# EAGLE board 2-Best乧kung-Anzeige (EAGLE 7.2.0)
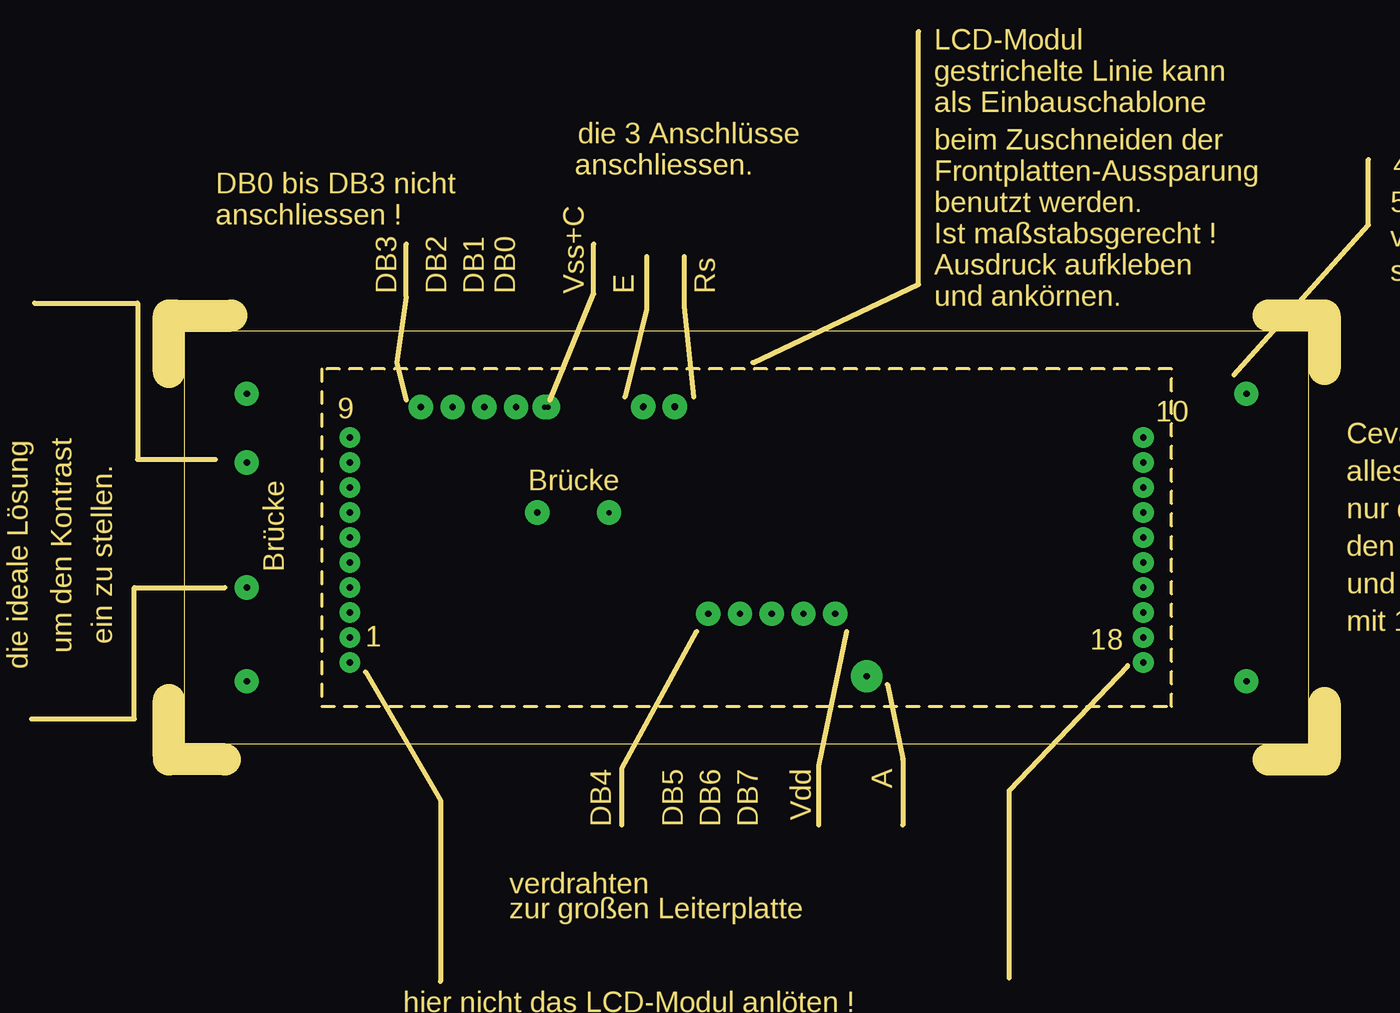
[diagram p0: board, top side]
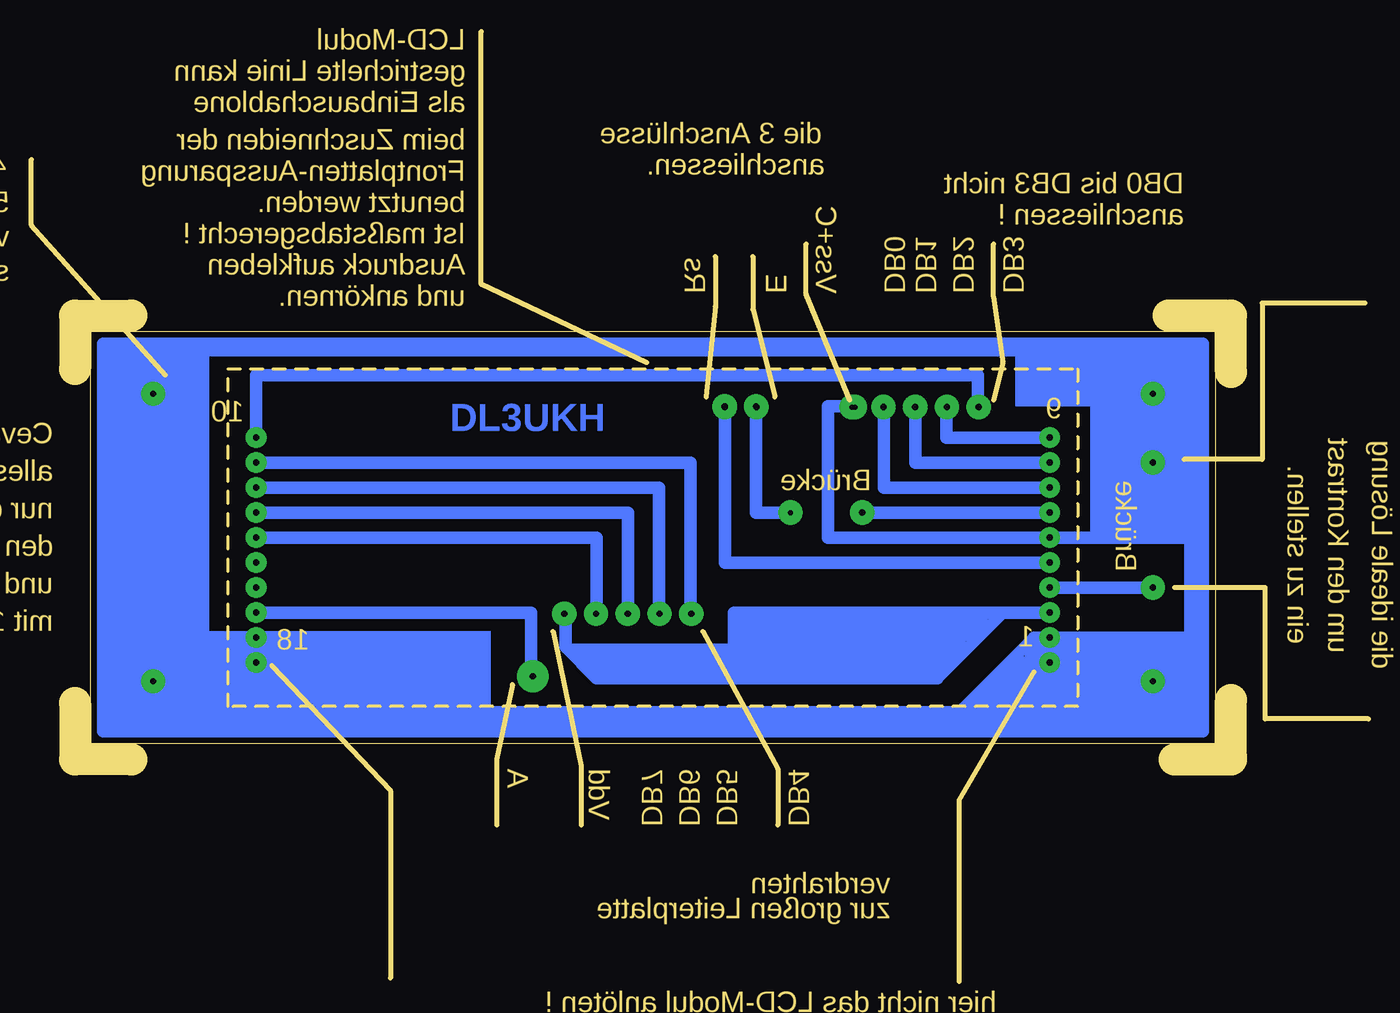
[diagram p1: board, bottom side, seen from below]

Size 107 x 76 mm. Coordinates in mm from the lower left corner, seen from the top.
Outline: 46 segments
Copper layers (1*16): Top 0.035mm / dielectric 1.5mm / Bottom 0.035mm
Design rules "default": minimum track width 10mil, minimum drill 24mil, track to track 8mil, track to pad 8mil, pad to pad 8mil, via to via 8mil, smd to smd 8mil, copper to edge 40mil, drill to drill 8mil, minimum pad ring 10mil, minimum via ring 8mil, stop-mask expansion 4mil, vias tented up to drill 0mil, thermal gap 10mil

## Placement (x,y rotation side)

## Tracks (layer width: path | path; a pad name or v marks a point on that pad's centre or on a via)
S$1  (via drill 0.4 pad 1.93)
  other vias: 17.25,24
S$2  (via drill 0.4 pad 1.68)
  Bottom 1.016: 31.75,21.5 27.75,25.5 v25.5,25.5 v25.5,27.5 26.75,27.5 33,21.25
S$3  (via drill 0.5 pad 1.68)
  Bottom 1.016: 31.75,21.5 27.75,25.5 v25.5,25.5 v25.5,27.5 26.75,27.5 33,21.25
S$4  (via drill 0.4 pad 1.93)
  other vias: 17.25,47
S$5  (via drill 0.4 pad 1.93)
  other vias: 97.25,24
S$6  (via drill 0.5 pad 1.68, 0.5 pad 1.93)
  Bottom 1.016: 54.25,29.5 54.25,41.5 v89,41.5
  other vias: 54.18,29.4
S$7  (via drill 0.5 pad 1.68)
  other vias: 25.5,31.5
S$8  (via drill 0.5 pad 1.93)
  other vias: 17.25,24
S$9  (via drill 0.4 pad 1.93)
  other vias: 97.25,47
S$10  (via drill 0.5 pad 1.93)
  other vias: 17.25,47
S$11  (via drill 0.5 pad 1.93)
  other vias: 97.25,24
S$12  (via drill 0.5 pad 1.93)
  other vias: 97.25,47
S$13
  Bottom 1.016: 93.25,20.25 93.25,51 98,51 | 21,51 21.25,51 | 21,51 98,51 | 98,51 101.25,51 101.25,20 13.25,20 13.25,51 21,51
S$14  (via drill 0.4 pad 1.68, 0.4 pad 1.93)
  Bottom 1.016: 17,31.5 v25.5,31.5 | 13.5,35.5 14.25,35.5 | 14.25,35.5 v25.5,35.5 43.25,35.5 43.25,46 41.25,46 | 31.75,21.5 27.75,25.5 v25.5,25.5 | 33,21.25 26.75,27.5 v25.5,27.5 | v25.5,25.5 20.5,25.5 | v25.5,27.5 v25.5,25.5 | 21.25,27.5 v25.5,27.5 | 21.25,27.5 14.25,27.5 | 14.25,27.5 13.75,27.5 | 21.25,20.25 21.25,27.5 | 14.25,35.5 14.25,27.5
  other vias: 41.34,45.94
S$15  (via drill 0.5 pad 1.68, 0.5 pad 1.93)
  Bottom 1.016: 56.75,29.5 56.75,39.5 v89,39.5
  other vias: 56.72,29.4
S$16  (via drill 0.4 pad 1.68)
  Bottom 1.016: v89,27.5 93.5,27.5
S$17  (via drill 0.4 pad 1.68)
  other vias: 89,31.5
S$18  (via drill 0.5 pad 1.68, 0.5 pad 1.93)
  Bottom 1.016: 59.25,29.5 59.25,37.5 v89,37.5
  other vias: 59.26,29.4
S$19  (via drill 0.5 pad 1.68, 0.5 pad 1.93)
  Bottom 1.016: 61.75,29.5 61.75,35.5 v89,35.5
  other vias: 61.8,29.4
S$20  (via drill 0.5 pad 1.68, 0.5 pad 1.93)
  Bottom 1.016: 31.25,45.75 31.25,48.5 35.75,48.5 | 35.75,48.5 36,48.5 | 35.75,48.5 89,48.5 v89,43.5
  other vias: 31.18,45.94
S$21  (via drill 0.5 pad 1.68)
  other vias: 25.5,31.5
S$22  (via drill 0.5 pad 1.93)
  other vias: 49,46 48.96,45.94
S$23  (via drill 0.4 pad 1.93)
  other vias: 17.25,24
S$24  (via drill 0.5 pad 1.68)
  other vias: 25.5,35.5
S$25  (via drill 0.4 pad 1.68)
  other vias: 89,33.5
S$26  (via drill 0.5 pad 1.93)
  other vias: 51.5,46 51.5,45.94
S$27  (via drill 0.5 pad 1.68, 0.5 pad 1.93)
  Bottom 1.016: v25.5,41.5 36.25,41.5 36.25,46
  other vias: 36.26,45.94
S$28  (via drill 0.5 pad 1.68)
  Bottom 1.016: v89,27.5 93.5,27.5
S$29  (via drill 0.5 pad 1.68)
  other vias: 89,31.5
S$30  (via drill 0.5 pad 1.68, 0.5 pad 1.93)
  Bottom 1.016: 38.75,46 38.75,39.5 v25.5,39.5
  other vias: 38.8,45.94
S$31  (via drill 0.5 pad 1.68)
  other vias: 89,33.5
S$32  (via drill 0.5 pad 1.68)
  other vias: 25.5,33.5
S$33  (via drill 0.5 pad 1.68, 0.5 pad 1.93)
  Bottom 1.016: 64.25,29.5 64.25,26.75 61.75,24.25 34.5,24.25 29.25,29.5 v25.5,29.5
  other vias: 64.34,29.4
S$34  (via drill 0.4 pad 1.93)
  other vias: 17.25,47
S$35  (via drill 0.5 pad 1.68, 0.5 pad 2.54)
  Bottom 1.016: 67,24.5 67,29.5 v89,29.5
  other vias: 66.86,24.4
S$36  (via drill 0.5 pad 1.68)
  other vias: 25.5,25.5
S$37  (via drill 0.5 pad 1.68)
  Bottom 1.016: v89,25.5 93.5,25.5
S$38  (via drill 0.5 pad 1.68, 0.5 pad 1.93)
  Bottom 1.016: v25.5,43.5 33.75,43.5 33.75,46
  other vias: 33.72,45.94
S$39  (via drill 0.5 pad 1.68, 0.5 pad 1.93)
  Bottom 1.016: v25.5,41.5 36.25,41.5 36.25,46
  other vias: 36.26,45.94
S$40  (via drill 0.5 pad 1.68, 0.5 pad 1.93)
  Bottom 1.016: 54.25,29.5 54.25,41.5 v89,41.5
  other vias: 54.18,29.4
S$41  (via drill 0.5 pad 1.68, 0.5 pad 1.93)
  Bottom 1.016: 56.75,29.5 56.75,39.5 v89,39.5
  other vias: 56.72,29.4
S$42  (via drill 0.5 pad 1.68, 0.5 pad 1.93)
  Bottom 1.016: 59.25,29.5 59.25,37.5 v89,37.5
  other vias: 59.26,29.4
S$43  (via drill 0.5 pad 1.68, 0.5 pad 1.93)
  Bottom 1.016: 61.75,29.5 61.75,35.5 v89,35.5
  other vias: 61.8,29.4
S$44  (via drill 0.5 pad 1.68, 0.5 pad 1.93)
  Bottom 1.016: 31.25,45.75 31.25,48.5 35.75,48.5 | 35.75,48.5 36,48.5 | 35.75,48.5 89,48.5 v89,43.5
  other vias: 31.18,45.94
S$45  (via drill 0.5 pad 1.68, 0.5 pad 1.93)
  Bottom 1.016: 38.75,46 38.75,39.5 v25.5,39.5
  other vias: 38.8,45.94
S$46  (via drill 0.5 pad 1.68, 0.5 pad 1.93)
  Bottom 1.016: 64.25,29.5 64.25,26.75 61.75,24.25 50.75,24.25 | 50.75,24.25 34.5,24.25 29.25,29.5 28.75,29.5 | 28.75,29.5 v25.5,29.5 | 28.75,29.5 50.75,29.5 50.75,24.25
  other vias: 64.34,29.4
S$47  (via drill 0.5 pad 1.68, 0.5 pad 2.54)
  Bottom 1.016: 67,24.5 67,29.5 v89,29.5
  other vias: 66.86,24.4
S$48  (via drill 0.5 pad 1.68)
  Bottom 1.016: v89,25.5 93.5,25.5
S$49  (via drill 0.5 pad 1.68, 0.5 pad 1.93)
  Bottom 1.016: v25.5,43.5 33.75,43.5 33.75,46
  other vias: 33.72,45.94
S$50  (via drill 0.5 pad 1.93)
  other vias: 49,46 48.96,45.94
S$51  (via drill 0.5 pad 1.93)
  Bottom 1.016: 51.5,34 v51.5,46
  other vias: 51.5,45.94
S$52  (via drill 0.4 pad 1.93)
  other vias: 97.25,24
S$53  (via drill 0.5 pad 1.68)
  other vias: 25.5,33.5 25.5,33.5
S$54  (via drill 0.5 pad 1.68)
  other vias: 25.5,37.5
S$55  (via drill 0.4 pad 1.93)
  other vias: 97.25,47
S$56
  Bottom 1.016: 93.25,20.25 93.25,51 98,51 | 21,51 21.25,51 | 21,51 98,51 | 98,51 101.25,51 101.25,20 13.25,20 13.25,51 21,51
S$57  (via drill 0.4 pad 1.68, 0.4 pad 1.93)
  Bottom 1.016: v25.5,35.5 43.25,35.5 43.25,46 41.25,46
  other vias: 25.5,31.5 41.09,45.94
S$58  (via drill 0.4 pad 1.68, 0.4 pad 1.93)
  Bottom 1.016: v25.5,41.5 36.25,41.5 36.25,46
  other vias: 36.26,45.94
S$59  (via drill 0.4 pad 1.68)
  Bottom 1.016: v89,27.5 93.5,27.5
S$60  (via drill 0.4 pad 1.68)
  other vias: 89,31.5
S$61  (via drill 0.4 pad 1.68)
  other vias: 89,33.5
S$62  (via drill 0.4 pad 1.68, 0.4 pad 1.93)
  Bottom 1.016: v25.5,41.5 36.25,41.5 36.25,46
  other vias: 36.26,45.94
S$63  (via drill 0.4 pad 1.68, 0.4 pad 1.93)
  Bottom 1.016: 54.25,29.5 54.25,41.5 v89,41.5
  other vias: 54.18,29.4
S$64  (via drill 0.4 pad 1.68, 0.4 pad 1.93)
  Bottom 1.016: 56.75,29.5 56.75,39.5 v89,39.5
  other vias: 56.72,29.4
S$65  (via drill 0.4 pad 1.68, 0.4 pad 1.93)
  Bottom 1.016: 59.25,29.5 59.25,37.5 v89,37.5
  other vias: 59.26,29.4
S$66  (via drill 0.4 pad 1.68, 0.4 pad 1.93)
  Bottom 1.016: 61.75,29.5 61.75,35.5 v89,35.5
  other vias: 61.8,29.4
S$67  (via drill 0.4 pad 1.68, 0.4 pad 1.93)
  Bottom 1.016: 31.25,45.75 31.25,48.5 35.75,48.5 | 35.75,48.5 36,48.5 | 35.75,48.5 89,48.5 v89,43.5
  other vias: 31.18,45.94
S$68  (via drill 0.4 pad 1.68, 0.4 pad 1.93)
  Bottom 1.016: 38.75,46 38.75,39.5 v25.5,39.5
  other vias: 38.8,45.94
S$69  (via drill 0.4 pad 1.68, 0.4 pad 1.93)
  Bottom 1.016: 64.25,29.5 64.25,26.75 61.75,24.25 50.75,24.25 | 50.75,24.25 34.5,24.25 29.25,29.5 28.75,29.5 | 28.75,29.5 v25.5,29.5 | 28.75,29.5 50.75,29.5 50.75,24.25
  other vias: 64.34,29.4
S$70  (via drill 0.4 pad 1.68, 0.4 pad 2.54)
  Bottom 1.016: 67,24.5 67,29.5 v89,29.5
  other vias: 66.86,24.4
S$71  (via drill 0.4 pad 1.68)
  Bottom 1.016: v89,25.5 93.5,25.5
S$72  (via drill 0.4 pad 1.68, 0.4 pad 1.93)
  Bottom 1.016: v25.5,43.5 33.75,43.5 33.75,46
  other vias: 33.72,45.94
S$73  (via drill 0.4 pad 1.93)
  Bottom 1.016: v46.25,37.5 49,37.5 49,46
  other vias: 48.96,45.94
S$74  (via drill 0.4 pad 1.68, 0.4 pad 1.93)
  Bottom 1.016: v25.5,33.5 51.5,33.5 51.5,46
  other vias: 51.5,45.94
S$75  (via drill 0.4 pad 1.68)
  Bottom 1.016: v25.5,33.5 33.75,33.5
S$76  (via drill 0.4 pad 1.68, 0.5 pad 1.93)
  Bottom 1.016: v25.5,37.5 v40.5,37.5
S$77  (via drill 0.4 pad 1.68, 0.4 pad 1.93)
  Bottom 1.016: 54.25,29.5 54.25,41.5 v89,41.5
  other vias: 54.18,29.4
S$78  (via drill 0.4 pad 1.68, 0.4 pad 1.93)
  Bottom 1.016: 56.75,29.5 56.75,39.5 v89,39.5
  other vias: 56.72,29.4
S$79  (via drill 0.4 pad 1.68, 0.4 pad 1.93)
  Bottom 1.016: 59.25,29.5 59.25,37.5 v89,37.5
  other vias: 59.26,29.4
S$80  (via drill 0.4 pad 1.68, 0.4 pad 1.93)
  Bottom 1.016: 61.75,29.5 61.75,35.5 v89,35.5
  other vias: 61.8,29.4
S$81  (via drill 0.4 pad 1.68, 0.4 pad 1.93)
  Bottom 1.016: 31.25,45.75 31.25,48.5 35.75,48.5 | 35.75,48.5 36,48.5 | 35.75,48.5 89,48.5 v89,43.5
  other vias: 31.18,45.94
S$82  (via drill 0.4 pad 1.68, 0.4 pad 1.93)
  Bottom 1.016: 38.75,46 38.75,39.5 v25.5,39.5
  other vias: 38.8,45.94
S$83  (via drill 0.4 pad 1.68, 0.4 pad 1.93)
  Bottom 1.016: 64.25,29.5 64.25,26.75 61.75,24.25 50.75,24.25 | 50.75,24.25 34.5,24.25 29.25,29.5 28.75,29.5 | 28.75,29.5 v25.5,29.5 | 28.75,29.5 50.75,29.5 50.75,24.25
  other vias: 64.34,29.4
S$84  (via drill 0.4 pad 1.68, 0.4 pad 2.54)
  Bottom 1.016: 67,24.5 67,29.5 v89,29.5
  other vias: 66.86,24.4
S$85  (via drill 0.4 pad 1.68)
  Bottom 1.016: v89,25.5 93.5,25.5
S$86  (via drill 0.4 pad 1.68, 0.4 pad 1.93)
  Bottom 1.016: v25.5,43.5 33.75,43.5 33.75,46
  other vias: 33.72,45.94
S$87  (via drill 0.4 pad 1.93)
  Bottom 1.016: v46.25,37.5 49,37.5 49,46
  other vias: 48.96,45.94
S$88  (via drill 0.4 pad 1.68, 0.4 pad 1.93)
  Bottom 1.016: v25.5,33.5 51.5,33.5 51.5,46
  other vias: 51.5,45.94
S$89  (via drill 0.4 pad 1.68)
  Bottom 1.016: v25.5,33.5 33.75,33.5
S$90  (via drill 0.4 pad 1.68, 0.5 pad 1.93)
  Bottom 1.016: v25.5,37.5 v40.5,37.5
S$91
  Bottom 1.016: 93.25,20.25 93.25,51 98,51 | 21,51 21.25,51 | 21,51 98,51 | 98,51 101.25,51 101.25,20 13.25,20 13.25,51 21,51
S$92  (via drill 0.5 pad 1.93)
  other vias: 17.25,31.5
S$93  (via drill 0.5 pad 1.93)
  other vias: 17.25,41.5
(copper drawn outside any net)
  shapes: Bottom area x22

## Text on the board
Bottom: DL3UKH
Vias: Auf Bestückungsseite gesehen ! | Es ist die selbe Leiterplatte wie aus 4-Basteleien | mit "Leiterplatte-Anzeige" !
Dimension: LCD-Modul | gestrichelte Linie kann | als Einbauschablone | die 3 Anschlüsse | beim Zuschneiden der | anschliessen. | 4 Stck. | Frontplatten-Aussparung | DB0 bis DB3 nicht | anschliessen ! | benutzt werden. | 5 mm Distanzbolzen | Ist maßstabsgerecht ! | verwendet man 2stck. Buchsenleisten | Ausdruck aufkleben | sollten es 10mm Distanzbolzen sein ! | DB3 | DB2 | DB1 | DB0 | Vss+C | E | Rs | und ankörnen. | 9 | 10 | Cevausit 1,5mm dick | alles mit 0,8mm gebohrt | Brücke | nur die Befestigungs-Bohrungen von | den Distanzbolzen mit 3,2mm bohren. | Brücke | und die Anschlüsse kann man | mit 1,0mm bohren. | ein zu stellen. | 1 | 18 | um den Kontrast | die ideale Lösung | Die Brücke war bisher | DB4 | DB5 | DB6 | DB7 | Vdd | A | verdrahten | zur großen Leiterplatte | hier nicht das LCD-Modul anlöten ! | nur oberhalb bei Buchse 1...9 und 10...18 ! | ODER : | 2 Stck. Buchsenleisten Raster 2,00mm x 10 Bestell Reichelt: 2stck. BL 1x10G 2,00 | 1stck. Buchsenleiste hat 10 Anschlüsse | und nicht nur 9, wie das LCD-Modu. Deshalb Achtung beim Reinstecken ! | Es ist besser man lötet das LCD-Modul direkt ein. Es fällt dann nicht aus den Buchsenleisten ! | BEI ROBUSTEM EINSATZ !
